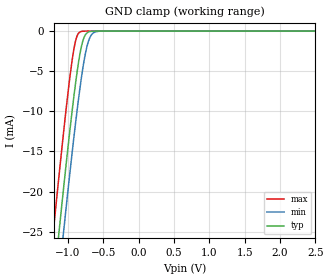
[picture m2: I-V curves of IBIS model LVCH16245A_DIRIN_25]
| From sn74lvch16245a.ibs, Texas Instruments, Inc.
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[Model]   LVCH16245A_DIRIN_25
Model_type  Input
Vinl=0.7
Vinh=1.7
| variable   typ   min   max
C_comp   2.72pF   2.12pF   3.55pF
[Temperature Range]   40   100   -40
| Ambient temperature   25   85   -40
[Voltage range]   2.5   2.3   2.7
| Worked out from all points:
|   GND clamp passes 1 mA (typ) near -0.78 V on its own axis
[GND Clamp]
| LVCH16245A_DIRIN_25
|   Voltage   I(typ)   I(min)   I(max)
-5V       -385.1mA   -389.7mA   -379.3mA
-1.205V   -31.84mA   -37.3mA    -24.82mA
-1.13V    -25.34mA   -30.81mA   -18.32mA
-1.07V    -20.26mA   -25.7mA    -13.28mA
-1.05V    -18.59mA   -24.02mA   -11.64mA
-955mV    -11mA      -16.27mA   -4.534mA
-885mV    -6.001mA   -10.91mA   -980.1uA
-830mV    -2.824mA   -7.089mA   -113.2uA
-780mV    -970.8uA   -4.107mA   -11.31uA
-710mV    -114.6uA   -1.265mA   -421.5nA
-645mV    -12.19uA   -255.7uA   -19.77nA
2.5V      4.712pA    6.752pA    4.389pA
